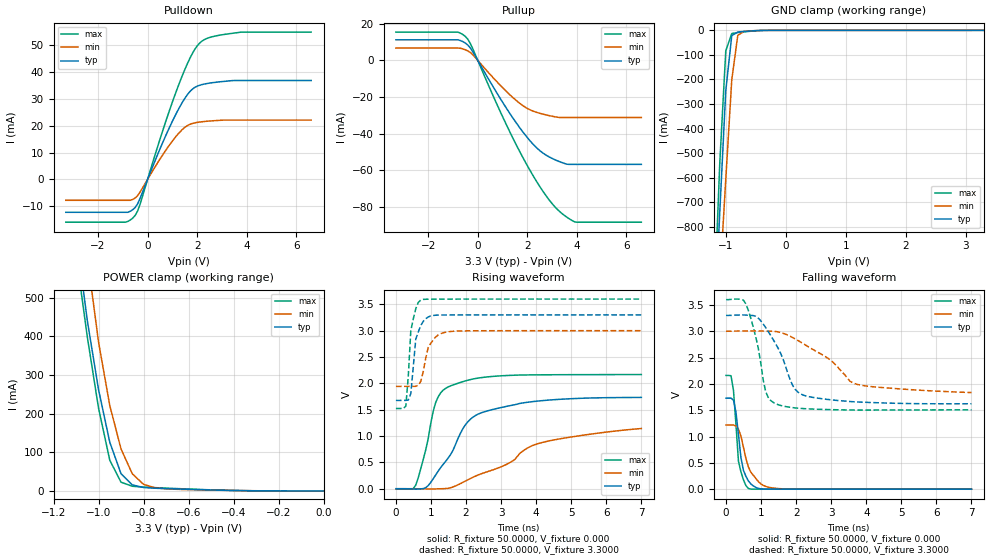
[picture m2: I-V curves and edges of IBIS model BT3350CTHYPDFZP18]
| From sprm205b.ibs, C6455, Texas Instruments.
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|   Model BT3350CTHYPDFZP18
[Model]   BT3350CTHYPDFZP18
Model_type   I/O
Polarity   Non-Inverting
Enable   Active-Low
Vinl =   0.8000V
Vinh =   2.0000V
Vmeas =   1.5000V
Cref =  10.0000pF
Rref =  50.0000
Vref =   1.5000V
C_comp   1.3646pF   1.3114pF   1.4331pF
[Temperature Range]   25.0000   0.1250k   -40.0000
[Pullup Reference]   3.3000V   3.0000V   3.6000V
[Pulldown Reference]   0.000V   0.000V   0.000V
[POWER Clamp Reference]   3.3000V   3.0000V   3.6000V
[GND Clamp Reference]   0.000V   0.000V   0.000V
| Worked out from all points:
|   slope of the pulldown table from 0 to 0.495 V, typ, clamps not added: 44 ohm
|   slope of the pullup table from 0 to 0.495 V, typ, clamps not added: 42.8 ohm
|   GND clamp passes 1 mA (typ) near -0.47 V on its own axis
|   POWER clamp passes 1 mA (typ) near -0.38 V on its own axis
|   rising waveform, R_fixture 50.0000, V_fixture 0.000: 20-80 % time 1.04ns typ, 2.18ns min, 468ps max; typ from 0 V to 1.73 V
|   rising waveform, R_fixture 50.0000, V_fixture 3.3000: 20-80 % time 186ps typ, 273ps min, 155ps max; typ from 1.68 V to 3.3 V
|   falling waveform, R_fixture 50.0000, V_fixture 0.000: 20-80 % time 208ps typ, 366ps min, 160ps max; typ from 1.73 V to 0 V
|   falling waveform, R_fixture 50.0000, V_fixture 3.3000: 20-80 % time 680ps typ, 1.32ns min, 374ps max; typ from 3.3 V to 1.62 V
[Pulldown]
| voltage   I(typ)   I(min)   I(max)
-3.3V     -12.32mA   -7.834mA   -16.01mA
-800mV    -12.32mA   NA         -15.72mA
-500mV    -10.49mA   -6.966mA   -13.46mA
-300mV    -7.034mA   -4.709mA   -9.192mA
600mV     13.53mA    9.001mA    17.88mA
1.3V      27.11mA    17.65mA    36.39mA
1.8V      33.62mA    20.84mA    46.89mA
2V        34.78mA    21.25mA    49.84mA
2.2V      35.39mA    21.5mA     51.66mA
2.6V      36.06mA    21.83mA    53.22mA
3.5V      36.9mA     NA         54.62mA
6.6V      36.9mA     22.12mA    54.98mA
[Pullup]
| voltage   I(typ)   I(min)   I(max)
-3.3V     11.22mA    6.704mA    15.43mA
-800mV    11.22mA    6.704mA    15.43mA
-500mV    9.447mA    5.764mA    13.06mA
-300mV    6.8mA      4.287mA    9.245mA
1V        -22.82mA   -14.89mA   -30.69mA
2V        -42.2mA    -26.29mA   -57.53mA
2.4V      -48.09mA   -28.51mA   -66.74mA
2.8V      -52.14mA   -29.95mA   -74.81mA
3.2V      -54.81mA   -31.05mA   -81.26mA
3.5V      -56.33mA   NA         -84.78mA
3.7V      -56.86mA   NA         -86.64mA
6.6V      -56.86mA   -31.24mA   -88.43mA
[GND_clamp]
| voltage   I(typ)   I(min)   I(max)
-3.3V     -15.87A    -14.34A    -17.08A
-1.2V     -1.264A    -1.455A    -1.162A
-1.1V     -739.6mA   -1.022A    -539.9mA
-1V       -245.3mA   -606.1mA   -83.38mA
-900mV    -21.36mA   -201mA     -13.01mA
-800mV    -6.972mA   -20.59mA   -8.88mA
-700mV    -4.638mA   -4.461mA   -6.333mA
-300mV    -39.49uA   -55.52uA   -61.83uA
3.3V      64nA       87.17uA    296.1nA
[POWER_clamp]
| voltage   I(typ)   I(min)   I(max)
-3.3V     13.83A     12.48A     14.95A
-1.1V     665.8mA    853.9mA    613.8mA
-1.05V    441.7mA    607.3mA    399.5mA
-1V       262.6mA    385.7mA    214.6mA
-950mV    126.1mA    221.3mA    79.57mA
-900mV    44.61mA    108.8mA    22.66mA
-850mV    15.61mA    44.43mA    12.1mA
-800mV    8.911mA    17.17mA    9.881mA
-750mV    7.015mA    8.23mA     8.52mA
-650mV    4.984mA    4.132mA    6.055mA
-350mV    700.6uA    797.9uA    623.7uA
0V        111.7nA    170.6nA    370.4nA
[Ramp]
| variable   typ   min   max
dV/dt_r   1.0400/1.0317n   0.6855/2.2296n   1.3003/0.4631n
dV/dt_f   1.0068/0.6733n   0.6990/1.3618n   1.2558/0.3701n
R_load = 50.0000
[Rising Waveform]
R_fixture = 50.0000
V_fixture = 0.000
V_fixture_min = 0.000
V_fixture_max = 0.000
| time   V(typ)   V(min)   V(max)
0s        44.33uV    36.2uV     84.24uV
565.7ps   -8.112mV   -204.5uV   69.16mV
848.5ps   19.24mV    -2.601mV   733.3mV
1.131ns   258.6mV    -3.246mV   1.632V
1.273ns   398.1mV    -631.5uV   1.817V
1.485ns   578.1mV    8.329mV    1.931V
1.98ns    1.212V     144.7mV    2.046V
2.546ns   1.465V     309.1mV    2.118V
4.101ns   1.668V     865.1mV    2.162V
7ns       1.733V     1.143V     2.167V
[Rising Waveform]
R_fixture = 50.0000
V_fixture = 3.3000
V_fixture_min = 3.0000
V_fixture_max = 3.6000
| time   V(typ)   V(min)   V(max)
0s        1.676V     1.942V     1.523V
282.8ps   1.677V     1.943V     1.569V
353.5ps   1.683V     1.943V     2.148V
424.2ps   1.806V     1.943V     2.996V
565.7ps   2.838V     1.944V     3.416V
707.1ps   3.096V     2.036V     3.581V
919.2ps   3.26V      2.677V     3.597V
1.131ns   3.293V     2.879V     3.599V
1.414ns   3.298V     2.97V      3.599V
7ns       3.3V       3V         3.6V
[Falling Waveform]
R_fixture = 50.0000
V_fixture = 0.000
V_fixture_min = 0.000
V_fixture_max = 0.000
| time   V(typ)   V(min)   V(max)
0s        1.728V     1.22V      2.16V
141.4ps   1.729V     1.22V      2.154V
212.1ps   1.69V      1.219V     1.875V
353.5ps   1.04V      1.141V     530.2mV
424.2ps   601.4mV    1.009V     330.3mV
494.9ps   360.3mV    798.6mV    180.3mV
636.4ps   156.8mV    422.6mV    13.15mV
989.9ps   6.284mV    102mV      777.2uV
1.414ns   763.7uV    16.65mV    339.5uV
7ns       8.3uV      76.74uV    17.29uV
[Falling Waveform]
R_fixture = 50.0000
V_fixture = 3.3000
V_fixture_min = 3.0000
V_fixture_max = 3.6000
| time   V(typ)   V(min)   V(max)
0s        3.3V       3V         3.6V
565.7ps   3.306V     3.005V     3.519V
848.5ps   3.282V     3.005V     2.889V
1.131ns   3.069V     3.001V     1.85V
1.414ns   2.762V     2.995V     1.624V
1.909ns   1.96V      2.876V     1.548V
2.263ns   1.773V     2.738V     1.528V
2.97ns    1.699V     2.455V     1.511V
3.748ns   1.656V     1.99V      1.502V
7ns       1.622V     1.835V     1.507V
